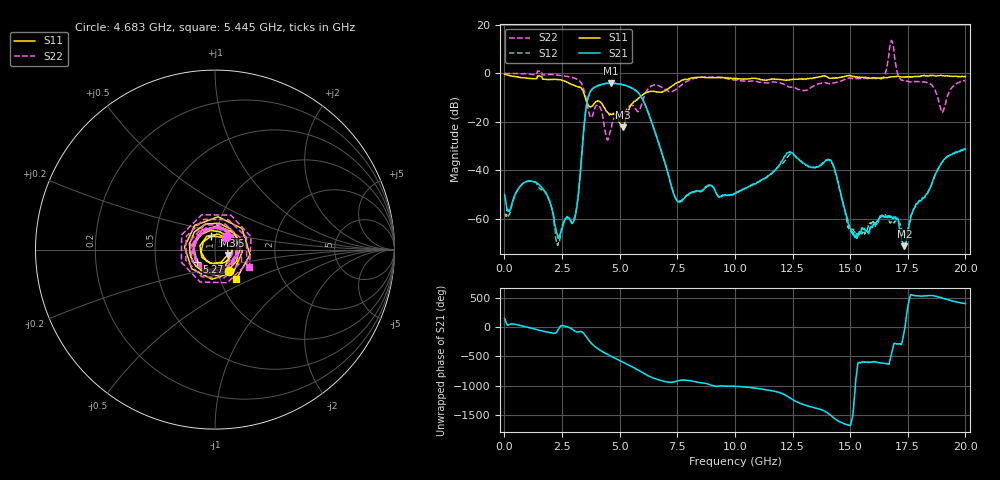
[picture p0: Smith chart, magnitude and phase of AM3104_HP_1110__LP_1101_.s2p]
!Created with skrf (http://scikit-rf.org).
# Hz S RI R 50.0
!freq ReS11 ImS11 ReS21 ImS21 ReS12 ImS12 ReS22 ImS22
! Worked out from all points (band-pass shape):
!   1601 points, 10 MHz to 20 GHz, reference 50 ohm
!   highest |S21| = -4.06 dB at 4.633 GHz (marker M1); lowest = -71.3 dB at 17.35 GHz (marker M2)
!   |S21| within 3 dB of the highest: 3.766 GHz to 5.693 GHz (1.928 GHz wide, 40.8 % of centre)
!   lowest |S11| = -22.3 dB at 5.132 GHz (marker M3), VSWR 1.17, Z = 57.5 - j3.5 ohm
!   |S11| at or under -10 dB: 3.507 GHz to 5.86 GHz (2.353 GHz wide, 50.2 % of centre)
!   |S22| runs from -27.5 to 13.5 dB; largest |S21 - S12| = 0.068
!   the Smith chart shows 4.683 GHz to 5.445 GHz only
!   S11 on the Smith chart (normalised r, x): 4.683 GHz: 1.14, -0.28; 5.095 GHz: 0.95, +0.14; 5.27 GHz: 0.81, -0.11; 5.445 GHz: 1.19, -0.41
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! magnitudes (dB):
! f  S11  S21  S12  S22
! 10 MHz  -0.4  -50.0  -58.1  -0.1
! 1.297 GHz  -2.3  -44.8  -44.7  -0.6
! 2.321 GHz  -2.6  -67.4  -70.9  -0.8
! 3.033 GHz  -5.1  -60.5  -59.5  -2.0
! 3.346 GHz  -6.3  -34.6  -34.7  -4.2
! 3.696 GHz  -13.7  -8.2  -8.3  -17.2
! 4.633 GHz  -16.9  -4.1  -4.2  -22.9
! 4.683 GHz  -16.8  -4.1  -4.2  -20.5
! 5.095 GHz  -22.1  -4.6  -4.7  -17.7
! 5.132 GHz  -22.3  -4.7  -4.7  -17.6
! 5.27 GHz  -18.5  -5.1  -5.1  -15.5
! 5.445 GHz  -13.8  -5.7  -5.7  -13.4
! 6.682 GHz  -7.8  -28.4  -28.4  -5.1
! 7.544 GHz  -3.7  -53.0  -52.7  -5.9
! 10.01 GHz  -2.3  -49.7  -49.7  -2.9
! 13.34 GHz  -2.2  -38.9  -38.8  -5.7
! 14.2 GHz  -2.1  -36.6  -36.9  -4.3
! 15.21 GHz  -1.5  -67.8  -65.7  -2.3
! 16.68 GHz  -1.6  -59.2  -60.7  7.2
! 17.35 GHz  -1.6  -71.3  -66.9  -3.2
! 19 GHz  -1.1  -36.6  -36.5  -16.2
! 20 GHz  -1.3  -31.2  -30.9  -3.0
